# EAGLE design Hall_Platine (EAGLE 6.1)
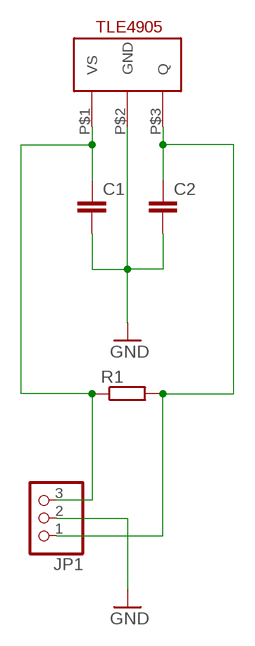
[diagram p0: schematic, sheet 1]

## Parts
C1  C-EUC0805  [C0805]
C2  C-EUC0805  [C0805]
JP1  PINHD-1X3  [1X03]
R1  R-EU_M0805  [M0805]
U$1  TLE4905  [TLE4905]

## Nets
GND: C1.2 C2.2 JP1.2 U$1.P$2(GND)
N$2: C1.1 JP1.3 R1.1 U$1.P$1(VS)
N$4: C2.1 JP1.1 R1.2 U$1.P$3(Q)

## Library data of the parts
C1 C2 = rcl:C-EU: CAPACITOR, European symbol
JP1 = pinhead:PINHD-1X3: PIN HEADER
R1 = rcl:R-EU_: RESISTOR, European symbol
U$1 = TLE4905:TLE4905

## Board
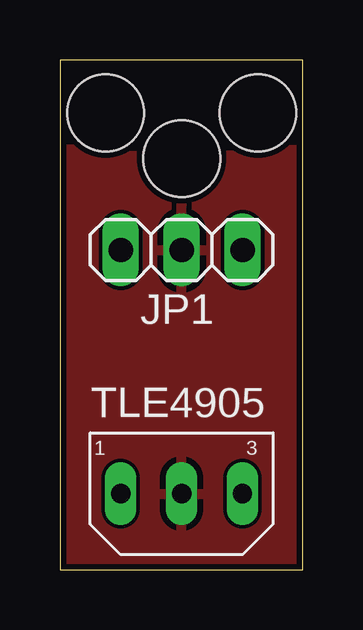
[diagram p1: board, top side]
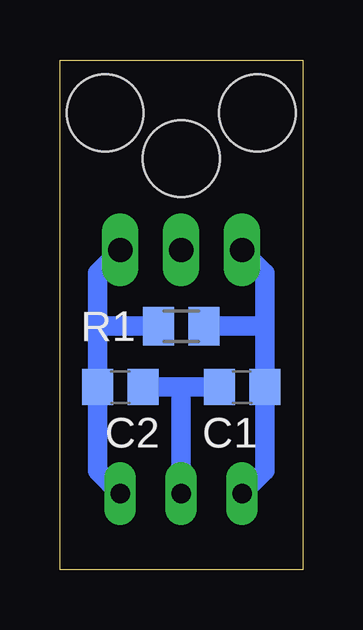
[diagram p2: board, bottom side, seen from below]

Size 10.14 x 21.26 mm. Coordinates in mm from the lower left corner, seen from the top.
Outline: 0,0 10.14,0 10.14,21.26 0,21.26 0,0
Copper layers (1*16): Top 0.035mm / dielectric 1.5mm / Bottom 0.035mm
Design rules: minimum track width 6mil, minimum drill 12mil, track to track 6mil, track to pad 6mil, pad to pad 6mil, via to via 6mil, smd to smd 0mil, copper to edge 10mil, drill to drill 10mil, minimum pad ring 10mil, minimum via ring 6mil, stop-mask expansion 2mil, vias tented up to drill 100mil, thermal gap 10mil
Holes 3.2 mm at 8.26,19.05 1.91,19.05 5.08,17.14

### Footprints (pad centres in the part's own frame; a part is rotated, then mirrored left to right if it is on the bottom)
C0805 = smd 1.3 x 1.5: 1 -0.95,0; 2 0.95,0
1X03 = drill 1.016 long: 1 -2.54,0; 2 0,0; 3 2.54,0
M0805 = smd 1.3 x 1.6: 1 -0.95,0; 2 0.95,0
TLE4905 = drill 0.8 long: P$1 0,0; P$2 -2.54,0; P$3 -5.08,0

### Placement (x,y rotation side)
C1  2.54,7.62 180 bottom
C2  7.62,7.62 0 bottom
JP1  5.08,13.34 180 top
R1  5.08,10.16 180 bottom
U$1  2.54,3.17 180 top

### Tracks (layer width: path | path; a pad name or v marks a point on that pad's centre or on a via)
GND
  Bottom 0.813: C1.2 5.08,7.62 | 5.08,7.62 C2.2 | U$1.P$2 5.08,7.62
  pour Top: -1.27,17.78 10.16,17.78 15.24,-1.27 -1.27,-1.27
N$2
  Bottom 0.813: U$1.P$1 1.59,4.13 C1.1 1.59,10.16 | 1.59,10.16 1.59,12.38 JP1.3 | R1.1 1.59,10.16
N$4
  Bottom 0.813: U$1.P$3 8.57,4.13 C2.1 8.57,10.16 | 8.57,10.16 8.57,12.38 JP1.1 | R1.2 8.57,10.16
